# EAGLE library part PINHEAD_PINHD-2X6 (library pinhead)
PIN HEADER
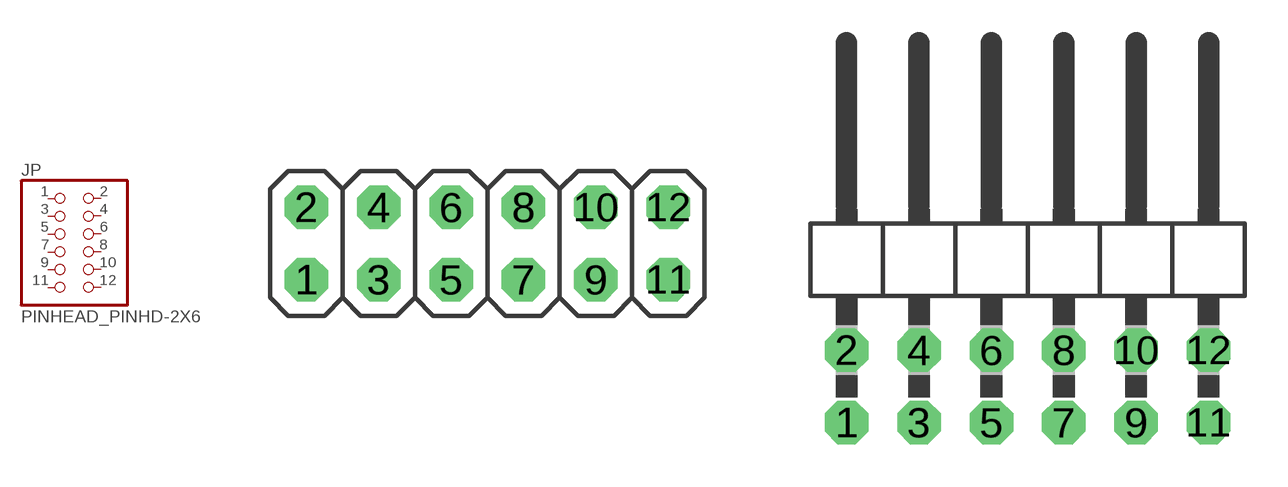
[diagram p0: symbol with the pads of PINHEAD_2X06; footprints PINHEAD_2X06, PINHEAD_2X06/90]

Designator prefix JP

## PINHEAD_PINHD-2X6  [PINHEAD_2X06]
1  1  pas
2  2  pas
3  3  pas
4  4  pas
5  5  pas
6  6  pas
7  7  pas
8  8  pas
9  9  pas
10  10  pas
11  11  pas
12  12  pas

## PINHEAD_PINHD-2X6/90  [PINHEAD_2X06/90]
Pads as for PINHEAD_2X06

## Footprint PINHEAD_2X06 (pad centres in mm)
PIN HEADER
drill 1.016 octagon: 1 -6.35,-1.27; 2 -6.35,1.27; 3 -3.81,-1.27; 4 -3.81,1.27; 5 -1.27,-1.27; 6 -1.27,1.27; 7 1.27,-1.27; 8 1.27,1.27; 9 3.81,-1.27; 10 3.81,1.27; 11 6.35,-1.27; 12 6.35,1.27

## Footprint PINHEAD_2X06/90 (pad centres in mm)
PIN HEADER
drill 1.016 octagon: 1 -6.35,-6.35; 2 -6.35,-3.81; 3 -3.81,-6.35; 4 -3.81,-3.81; 5 -1.27,-6.35; 6 -1.27,-3.81; 7 1.27,-6.35; 8 1.27,-3.81; 9 3.81,-6.35; 10 3.81,-3.81; 11 6.35,-6.35; 12 6.35,-3.81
